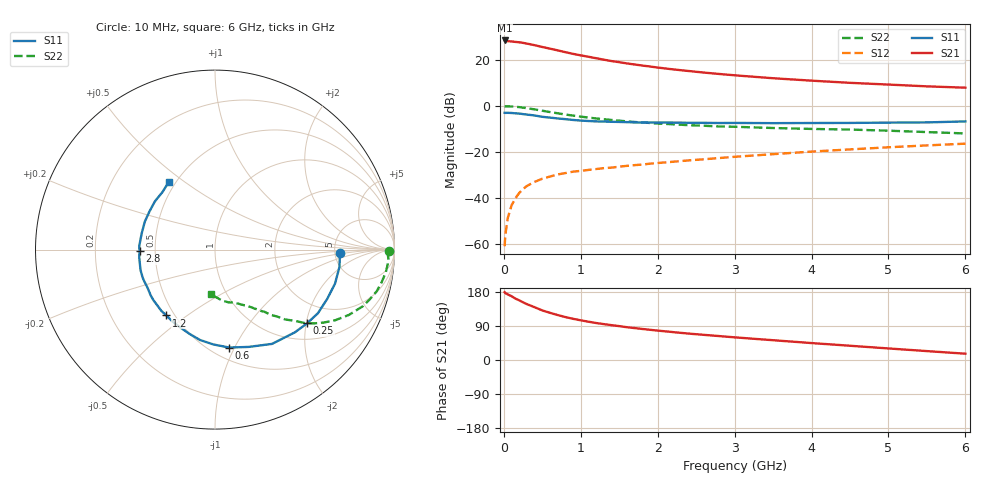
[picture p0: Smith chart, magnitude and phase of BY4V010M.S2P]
! SIEMENS Small Signal Semiconductors
! BFY420
! Si NPN RF SIEGET Grounded Emitter Transistor in MICRO-X
! VCE = 4 V  IC = 10 mA
! Common Emitter S-Parameters:  October  1996
# GHz  S  MA  R  50
!  f  S11  S21  S12  S22
! GHz  MAG  ANG  MAG  ANG  MAG  ANG  MAG  ANG
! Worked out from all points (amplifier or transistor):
!   36 points, 10 MHz to 6 GHz, reference 50 ohm
!   highest |S21| = 28.3 dB at 10 MHz (marker M1)
!   |S21| within 3 dB of that: start of sweep to 522.4 MHz
!   unconditionally stable (mu >= 1): start of sweep to 14.12 MHz; 2.516 GHz to end of sweep
!   at 250 MHz: K = 0.26, MSG = 31.7 dB, |S12| = -36.1 dB
!   at 1.4 GHz: K = 0.75, MSG = 23.1 dB, |S12| = -26.9 dB
!   at 6 GHz: K = 1.08, MAG = 10.4 dB, |S12| = -16.5 dB
!   S11 on the Smith chart (normalised r, x): 10 MHz: 5.61, -0.46; 250 MHz: 1.40, -2.02; 600 MHz: 0.61, -0.95; 1.2 GHz: 0.45, -0.42; 2.8 GHz: 0.41, -0.01; 6 GHz: 0.46, +0.43
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0.01  0.6991 -1.7  25.94 178.9  0.0009 28.9  0.9694 -0.6
0.02  0.697 -3.2  25.52 176.5  0.0016 62.6  0.9623 -1.2
0.05  0.7 -8.1  24.98 173.2  0.0036 69.9  0.969 -3.6
0.1  0.695 -15.9  24.71 168.4  0.0069 72.2  0.9603 -7.5
0.15  0.6827 -23.8  24.11 162.0  0.0098 72.3  0.9461 -11.1
0.2  0.6742 -31.7  23.67 157.5  0.0128 72.9  0.9308 -14.4
0.25  0.6573 -38.7  22.99 152.1  0.0156 67.8  0.9065 -17.7
0.3  0.6408 -46.0  22.18 147.4  0.0182 67.8  0.8839 -20.8
0.4  0.6141 -58.8  20.49 139.3  0.0223 62.4  0.8303 -26.0
0.5  0.5738 -70.9  18.7 130.8  0.0261 59.9  0.7773 -30.4
0.6  0.5512 -81.8  17.23 124.5  0.0291 57.1  0.7276 -34.0
0.8  0.5105 -99.4  14.45 113.3  0.0346 53.0  0.6435 -39.4
0.9  0.4904 -106.9  13.28 108.7  0.0371 52.1  0.6083 -41.1
1.1  0.4654 -120.7  11.49 101.1  0.0405 51.3  0.5526 -44.8
1.2  0.4561 -126.5  10.68 97.6  0.0423 51.2  0.5281 -46.1
1.6  0.4398 -144.7  8.239 86.5  0.0496 49.7  0.4565 -50.7
2.2  0.4305 -164.6  6.118 73.6  0.0609 49.6  0.3952 -56.2
2.8  0.4207 -178.7  4.872 63.1  0.0733 48.3  0.3541 -61.2
3.5  0.4183 167.3  3.935 52.2  0.0889 45.7  0.328 -66.7
4.5  0.4226 149.6  3.128 37.6  0.1127 40.1  0.3034 -75.6
5.5  0.4341 132.4  2.624 23.5  0.1377 32.7  0.2677 -87.8
6  0.4558 124.6  2.455 16.6  0.1501 28.7  0.25 -95.5
